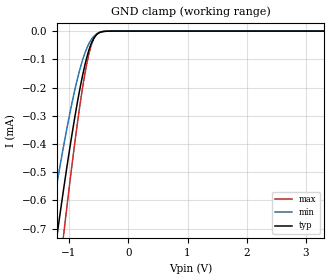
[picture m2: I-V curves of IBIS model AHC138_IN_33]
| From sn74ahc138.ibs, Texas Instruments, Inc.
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[Model]   AHC138_IN_33
Model_type  Input
Vinl=0.9
Vinh=2.1
| variable   typ   min   max
C_comp   0.91pF   0.80pF   0.99pF
[Temperature Range]   40   100   -40
| Ambient temperature   25   85   -40
[Voltage range]   3.3   3   3.6
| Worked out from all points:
|   GND clamp passes 1 mA (typ) near -1.38 V on its own axis
[GND Clamp]
| AHC138_IN_33
|   Voltage   I(typ)   I(min)   I(max)
-3.3V     -4.463mA   -3.643mA   -5.247mA
-1.365V   -975.1uA   -742.8uA   -1.237mA
-1.325V   -912uA     -691.3uA   -1.16mA
-1.205V   -727.2uA   -541.3uA   -931.7uA
-1.17V    -674.8uA   -499uA     -866.3uA
-1.08V    -543.4uA   -393.8uA   -701.3uA
-885mV    -283.6uA   -192.6uA   -367.4uA
-740mV    -127.5uA   -82.68uA   -160.9uA
-625mV    -43.98uA   -30.44uA   -50.86uA
-565mV    -19.84uA   -15.07uA   -20.7uA
-505mV    -7.613uA   -6.114uA   -6.771uA
3.3V      1.837nA    303.9pA    8.84nA
